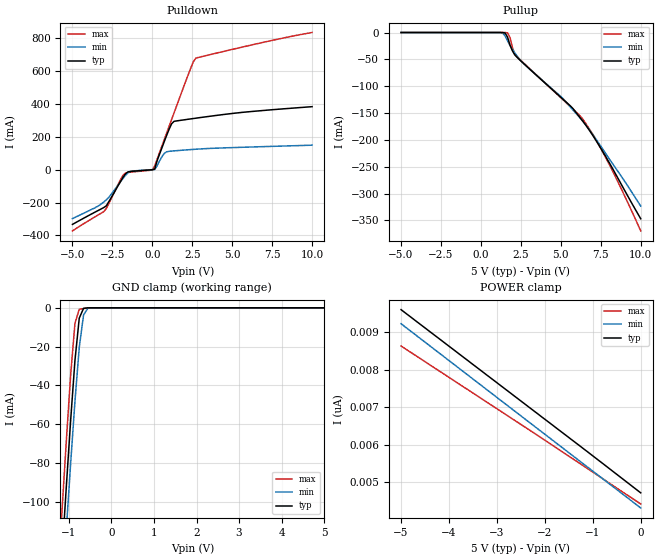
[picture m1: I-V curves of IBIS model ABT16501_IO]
|   TEXAS INSTRUMENTS INCORPORATED
|   Advanced Bus Logic Group
|   IBIS Model of SN74ABT16501
|   18-BIT UNIVERSAL BUS TRANSCEIVERS WITH 3-STATE OUTPUTS
|   56-pin DGG,DL Package
[IBIS Ver]   2.1
[Comment char]  |_char
[File Name]   abt16501.ibs
[File Rev]   2.0
[Date]   09/15/96
[Source]   File originated at Texas Instruments Incorporated.
[Notes]   The following is a sample IBIS file for the ABT16501.
   - This file may be incomplete or may not be fully compliant
   with the IBIS specification. It will be replaced with a
   version that is IBIS Revision 3.2 compliant and is complete
   and accurate. Please email all questions and comments to
   sllibis@ti.com.
|   - All test data contained in this file are derived from
|   hspice(tm) simulations.
|   - File created by Tareq Shahwan, ABL Applications
   - Disclaimer modified by David Holmgreen, Launch Marketing
[Disclaimer] Property of Texas Instruments Incorporated.  Unauthorized
   reproduction and/or distribution is strictly prohibited.
   This product is protected under copyright law.
   Created 1996, (C) Copyright 1996, Texas Instruments
   Incorporated, All Rights Reserved
   UNLESS THERE IS A SIGNED, WRITTEN AGREEMENT TO THE
   CONTRARY, TEXAS INSTRUMENTS ("TI") IS PROVIDING THE IBIS
   MODELS "AS IS" AND WITHOUT ANY WARRANTY, EXPRESSED OR
   IMPLIED.  TI assumes no liability for:
   1) the accuracy of the IBIS models provided to your
   company;
   2) the proper functioning of these IBIS models in your
   design or for any resulting applications; or
   3) infringement of patents, copyrights or intellectual
   property rights resulting from your use of these IBIS
   models.
   TI provides IBIS Models as a service to our customers.
   You and your company shall not distribute, sell or give
   these models to anyone else without prior written
   permission from TI.
   TI reserves the right to make changes to our products or
   to discontinue any semiconductor product or service
   without notice, and advises our customers to obtain the
   latest version of relevant information to verify, before
   placing orders, that the information being relied on is
   current.
   Please be aware that your receipt and use of the IBIS
   information provided shall serve as acceptance of these
   terms and conditions.  If you do not accept these terms,
   you should return or destroy the IBIS models and any
   other accompanying information immediately.
|   TSSOP   PACKAGE   (DGG)
[Component]   ABT16501_DGG
[manufacturer]   Texas Instruments Incorporated
[Package]
|   typ   min   max
R_pkg   0.045   0.035   0.062
L_pkg   3.324nH   2.403nH   5.094nH
C_pkg   0.564pF   0.341pF   0.914nH
[Pin]   signal_name   model_name   R_pin   L_pin   C_pin
1   OEAB   NC   0.062   5.094nH   0.856pF
2   LEAB   NC   0.061   4.621nH   0.902pF
3   A1   ABT16501_IO   0.06   4.316nH   0.802pF
4   GND   GND   0.059   3.968nH   0.698pF
5   A2   ABT16501_IO   0.057   3.716nH   0.649pF
6   A3   ABT16501_IO   0.042   3.517nH   0.652pF
7   VCC   POWER   0.041   3.16nH   0.57pF
8   A4   ABT16501_IO   0.039   2.981nH   0.482pF
9   A5   ABT16501_IO   0.039   2.809nH   0.447pF
10   A6   ABT16501_IO   0.038   2.715nH   0.409pF
11   GND   GND   0.041   2.675nH   0.391pF
12   A7   ABT16501_IO   0.039   2.536nH   0.366pF
13   A8   ABT16501_IO   0.039   2.457nH   0.348pF
14   A9   ABT16501_IO   0.038   2.411nH   0.353pF
15   A10   ABT16501_IO   0.039   2.456nH   0.355pF
16   A11   ABT16501_IO   0.039   2.471nH   0.349pF
17   A12   ABT16501_IO   0.04   2.58nH   0.37pF
18   GND   GND   0.038   2.651nH   0.389pF
19   A13   ABT16501_IO   0.038   2.739nH   0.411pF
20   A14   ABT16501_IO   0.039   2.838nH   0.449pF
21   A15   ABT16501_IO   0.038   2.988nH   0.484pF
22   VCC   POWER   0.038   3.105nH   0.564pF
23   A16   ABT16501_IO   0.04   3.427nH   0.638pF
24   A17   ABT16501_IO   0.056   3.654nH   0.641pF
25   GND   GND   0.057   3.932nH   0.7pF
26   A18   ABT16501_IO   0.058   4.257nH   0.806pF
27   OEBA_BAR   NC   0.057   4.58nH   0.914pF
28   LEBA   NC   0.059   5.038nH   0.861pF
29   GND   GND   0.06   5.058nH   0.858pF
30   CLKBA   NC   0.056   4.543nH   0.904pF
31   B18   ABT16501_IO   0.057   4.24nH   0.803pF
32   GND   GND   0.057   3.929nH   0.7pF
33   B17   ABT16501_IO   0.056   3.616nH   0.637pF
34   B16   ABT16501_IO   0.037   3.368nH   0.64pF
35   VCC   POWER   0.036   3.024nH   0.563pF
36   B15   ABT16501_IO   0.035   2.876nH   0.474pF
37   B14   ABT16501_IO   0.035   2.745nH   0.444pF
38   B13   ABT16501_IO   0.037   2.683nH   0.405pF
39   GND   GND   0.038   2.603nH   0.382pF
40   B12   ABT16501_IO   0.038   2.51nH   0.362pF
41   B11   ABT16501_IO   0.036   2.412nH   0.341pF
42   B10   ABT16501_IO   0.038   2.416nH   0.349pF
43   B9   ABT16501_IO   0.037   2.403nH   0.349pF
44   B8   ABT16501_IO   0.037   2.429nH   0.341pF
45   B7   ABT16501_IO   0.036   2.482nH   0.358pF
46   GND   GND   0.037   2.615nH   0.381pF
47   B6   ABT16501_IO   0.035   2.669nH   0.402pF
48   B5   ABT16501_IO   0.036   2.763nH   0.442pF
49   B4   ABT16501_IO   0.036   2.942nH   0.478pF
50   VCC   POWER   0.035   3.053nH   0.564pF
51   B3   ABT16501_IO   0.036   3.409nH   0.641pF
52   B2   ABT16501_IO   0.058   3.698nH   0.641pF
53   GND   GND   0.059   3.975nH   0.697pF
54   B1   ABT16501_IO   0.061   4.327nH   0.802pF
55   CLKAB   NC   0.061   4.624nH   0.905pF
56   GND   GND   0.06   5.063nH   0.858pF
|   SSOP   PACKAGE   (DL)
[Component]   ABT16501_DL
[manufacturer]   Texas Instruments Incorporated
[Package]
|   typ   min   max
R_pkg   0.055   0.048   0.067
L_pkg   6.539nH   4.802nH   9.746nH
C_pkg   0.85pF   0.5pF   1.351pF
[Pin]   signal_name   model_name   R_pin   L_pin   C_pin
1   OEAB   NC   0.064   9.646nH   1.202pF
2   LEAB   NC   0.059   8.723nH   1.348pF
3   A1   ABT16501_IO   0.059   8.139nH   1.223pF
4   GND   GND   0.056   7.554nH   1.088pF
5   A2   ABT16501_IO   0.054   6.991nH   0.966pF
6   A3   ABT16501_IO   0.053   6.659nH   0.973pF
7   VCC   POWER   0.055   6.321nH   0.905pF
8   A4   ABT16501_IO   0.055   5.942nH   0.713pF
9   A5   ABT16501_IO   0.057   5.767nH   0.678pF
10   A6   ABT16501_IO   0.054   5.459nH   0.631pF
11   GND   GND   0.051   5.224nH   0.638pF
12   A7   ABT16501_IO   0.048   5.088nH   0.601pF
13   A8   ABT16501_IO   0.05   5.021nH   0.518pF
14   A9   ABT16501_IO   0.051   4.802nH   0.5pF
15   A10   ABT16501_IO   0.051   4.803nH   0.5pF
16   A11   ABT16501_IO   0.05   5.021nH   0.518pF
17   A12   ABT16501_IO   0.048   5.088nH   0.601pF
18   GND   GND   0.051   5.224nH   0.638pF
19   A13   ABT16501_IO   0.054   5.459nH   0.631pF
20   A14   ABT16501_IO   0.057   5.768nH   0.677pF
21   A15   ABT16501_IO   0.055   5.942nH   0.715pF
22   VCC   POWER   0.055   6.321nH   0.907pF
23   A16   ABT16501_IO   0.053   6.659nH   0.972pF
24   A17   ABT16501_IO   0.054   6.991nH   0.966pF
25   GND   GND   0.056   7.554nH   1.087pF
26   A18   ABT16501_IO   0.059   8.139nH   1.223pF
27   OEBA_BAR   NC   0.059   8.727nH   1.351pF
28   LEBA   NC   0.067   9.746nH   1.21pF
29   GND   GND   0.063   9.63nH   1.203pF
30   CLKBA   NC   0.06   8.751nH   1.349pF
31   B18   ABT16501_IO   0.06   8.184nH   1.224pF
32   GND   GND   0.056   7.543nH   1.087pF
33   B17   ABT16501_IO   0.054   7.005nH   0.969pF
34   B16   ABT16501_IO   0.056   6.714nH   0.975pF
35   VCC   POWER   0.058   6.384nH   0.909pF
36   B15   ABT16501_IO   0.057   5.976nH   0.717pF
37   B14   ABT16501_IO   0.057   5.743nH   0.677pF
38   B13   ABT16501_IO   0.055   5.469nH   0.631pF
39   GND   GND   0.055   5.328nH   0.644pF
40   B12   ABT16501_IO   0.052   5.189nH   0.606pF
41   B11   ABT16501_IO   0.052   5.053nH   0.519pF
42   B10   ABT16501_IO   0.052   4.825nH   0.502pF
43   B9   ABT16501_IO   0.054   4.896nH   0.506pF
44   B8   ABT16501_IO   0.052   5.093nH   0.521pF
45   B7   ABT16501_IO   0.051   5.179nH   0.608pF
46   GND   GND   0.054   5.314nH   0.645pF
47   B6   ABT16501_IO   0.055   5.511nH   0.632pF
48   B5   ABT16501_IO   0.057   5.77nH   0.677pF
49   B4   ABT16501_IO   0.055   5.956nH   0.716pF
50   VCC   POWER   0.055   6.32nH   0.905pF
51   B3   ABT16501_IO   0.052   6.621nH   0.968pF
52   B2   ABT16501_IO   0.053   6.974nH   0.966pF
53   GND   GND   0.057   7.571nH   1.089pF
54   B1   ABT16501_IO   0.057   8.097nH   1.219pF
55   CLKAB   NC   0.059   8.723nH   1.349pF
56   GND   GND   0.061   9.56nH   1.199pF
| Models and submodels in the file (1): ABT16501_IO (I/O)
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|   Model ABT16501__IO
[Model]   ABT16501_IO
Model_type   I/O
Polarity   Inverting
Enable   Active-Low
Vinl = 0.8V
Vinh = 2.0V
|   typ   min   max
C_comp   7.46pF   NA   NA
[Temperature Range]   25   -40   85
[Voltage range]   5.0   4.5   5.5
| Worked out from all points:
|   slope of the pulldown table from 0 to 0.75 V, typ, clamps not added: 4.38 ohm
|   GND clamp passes 1 mA (typ) near -0.67 V on its own axis
[Pullup]   | Vtable = Vcc - Voutput
|Voltage   I(typ)   I(min)   I(max)
-5V       7.825nA    7.769nA    5.963nA
1.212V    -3.61uA    -124.9uA   -15.09nA
1.515V    -1.115mA   -6.541mA   -16.19uA
1.667V    -8.743mA   -15.51mA   -638.4uA
1.818V    -23.51mA   -24.23mA   -9.259mA
2.121V    -41.83mA   -37.99mA   -40.73mA
2.576V    -55.19mA   -54.99mA   -54.08mA
5V        -120.8mA   -119.3mA   -121.5mA
5.606V    -137mA     -139.1mA   -138.5mA
6.515V    -170.8mA   -170.4mA   -167.4mA
7.879V    -234.8mA   -228.7mA   -237mA
10V       -347.1mA   -323.5mA   -369.6mA
[Pulldown]
|Voltage   I(typ)   I(min)   I(max)
-5V       -332.7mA   -297.9mA   -371.9mA
-3.03V    -230.1mA   -196.5mA   -254.7mA
-1.97V    -68.89mA   -71.8mA    -57.5mA
-1.667V   -24.58mA   -33.86mA   -20.72mA
-1.364V   -11.59mA   -11.03mA   -15.87mA
0V        -1.216mA   -709.9uA   -2.502mA
151.5mV   3.142mA    234.2uA    22.68mA
757.6mV   171.8mA    98.51mA    184.5mA
1.212V    278.1mA    111.9mA    304.6mA
2.424V    307.2mA    121.1mA    619.5mA
2.727V    311.3mA    123.1mA    675.6mA
10V       381.1mA    147.6mA    830.8mA
[POWER_Clamp]   | Vtable = Vcc - Voutput
|Voltage   I(typ)   I(min)   I(max)
-5V       9.602nA    9.227nA    8.633nA
-2.172V   6.848nA    6.449nA    6.268nA
-1.111V   5.815nA    5.407nA    5.367nA
0V        4.719nA    4.315nA    4.422nA
[GND_Clamp]
|Voltage   I(typ)   I(min)   I(max)
-5V       -1.827A    -1.805A    -1.853A
-1.162V   -127.1mA   -149mA     -104mA
-1.061V   -91.81mA   -114mA     -68.2mA
-959.6mV  -57.91mA   -80.16mA   -34.59mA
-858.6mV  -27.06mA   -48.18mA   -7.95mA
-757.6mV  -5.332mA   -20.45mA   -772.3uA
-656.6mV  -272uA     -3.673mA   -365uA
-555.6mV  -10.37uA   -255.7uA   -142.8uA
5V        4.719nA    4.807nA    3.996nA
[Ramp]
|Variable   typ   min   max
dV/dt_r   1.511/0.570n   1.319/0.935n   1.683/0.724n
dV/dt_f   2.727/1.584n   2.340/2.602n   3.031/1.139n
